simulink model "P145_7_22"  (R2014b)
settings: Solver=ode45  StartTime=0.0  StopTime=10e-3  RelTol=1e-3
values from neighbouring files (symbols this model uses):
  E = (0:1/2:5)'    [IEDummyEx.m]    (also in Test01.m = sum((ObDat-y).^2); TestRtd02.m = sum((ObDat-y).^2))
  R = 1e3    (= 1000)    [IEDummyEx.m]
undefined symbols (not defined in the file or in its folder): C, L

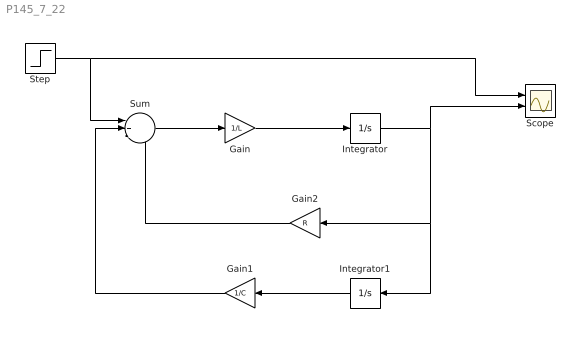
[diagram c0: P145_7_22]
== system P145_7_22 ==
  Gain : Gain  Gain=1/L
  Gain1 : Gain  Gain=1/C
  Gain2 : Gain  Gain=R
  Integrator : Integrator
  Integrator1 : Integrator
  Scope : Scope  NumInputPorts=2
  Step : Step  Time=0.001  After=E  SampleTime=0.00001
  Sum : Sum  Inputs=|+--
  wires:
  Step/1 -> Sum/1, Scope/1
  Sum/1 -> Gain/1
  Gain/1 -> Integrator/1
  Integrator/1 -> Integrator1/1, Gain2/1, Scope/2
  Integrator1/1 -> Gain1/1
  Gain1/1 -> Sum/2
  Gain2/1 -> Sum/3
